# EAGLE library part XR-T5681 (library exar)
2 MBPS PCM TRANSCEIVER
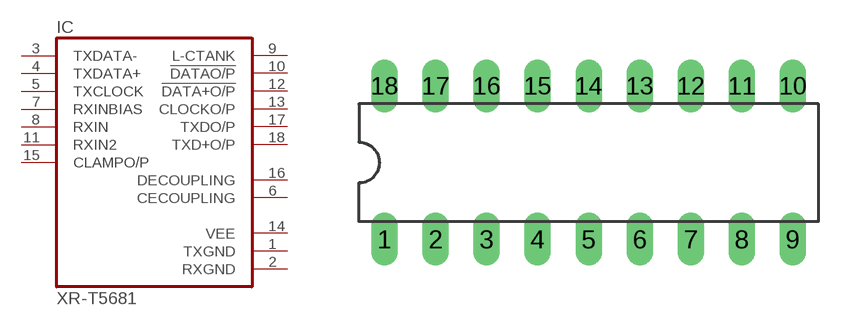
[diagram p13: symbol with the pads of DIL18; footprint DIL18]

Designator prefix IC

## XR-T5681 (OC_FARNELL: unknown; OC_NEWARK: unknown)  [DIL18]
1  TXGND  pwr
2  RXGND  pwr
3  TXDATA-  in
4  TXDATA+  in
5  TXCLOCK  in
6  CECOUPLING  out
7  RXINBIAS  in
8  RXIN  in
9  L-CTANK  out
10  !DATAO/P  out
11  RXIN2  in
12  !DATA+O/P  out
13  CLOCKO/P  out
14  VEE  pwr
15  CLAMPO/P  in
16  DECOUPLING  out
17  TXDO/P  out
18  TXD+O/P  out

## Footprint DIL18 (pad centres in mm)
Dual In Line Package
drill 0.813 long: 1 -10.16,-3.81; 2 -7.62,-3.81; 3 -5.08,-3.81; 4 -2.54,-3.81; 5 0,-3.81; 6 2.54,-3.81; 7 5.08,-3.81; 8 7.62,-3.81; 9 10.16,-3.81; 10 10.16,3.81; 11 7.62,3.81; 12 5.08,3.81; 13 2.54,3.81; 14 0,3.81; 15 -2.54,3.81; 16 -5.08,3.81; 17 -7.62,3.81; 18 -10.16,3.81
